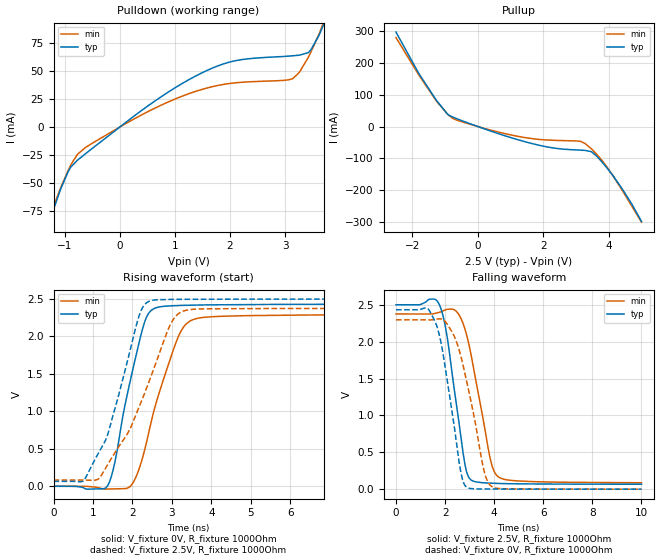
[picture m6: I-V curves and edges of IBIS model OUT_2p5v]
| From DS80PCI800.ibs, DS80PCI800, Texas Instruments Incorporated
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[Model]   OUT_2p5v
Model_type   Output
Polarity   Non-Inverting
Vmeas = 1.25
Vref = 0
Cref = 1pF
Rref = 1000000
|   typ   min   max
C_comp   1.378pF   1.280pF   1.479p
[Voltage Range]   2.5   2.375   2.625
[Temperature Range]   25   105   -40
[Pullup Reference]   2.5   2.375   2.625
[Pulldown Reference]   0   0   0
[Power Clamp Reference]   2.5   2.375   2.625
[GND Clamp Reference]   0   0   0
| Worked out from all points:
|   slope of the pulldown table from 0 to 0.375 V, typ, clamps not added: 26.8 ohm
|   slope of the pullup table from 0 to 0.375 V, typ, clamps not added: 27.5 ohm
|   falling waveform, V_fixture 2.5V, R_fixture 1000Ohm: 20-80 % time 601ps typ, 762ps min, NA max; typ from 2.5 V to 0.067 V
|   rising waveform, V_fixture 0V, R_fixture 1000Ohm: 20-80 % time 565ps typ, 749ps min, NA max; typ from 0 V to 2.43 V
|   rising waveform, V_fixture 2.5V, R_fixture 1000Ohm: 20-80 % time 777ps typ, 1.11ns min, NA max; typ from 0.065 V to 2.5 V
|   falling waveform, V_fixture 0V, R_fixture 1000Ohm: 20-80 % time 664ps typ, 842ps min, NA max; typ from 2.43 V to 0 V
[Pulldown]
|   Voltage   I(typ)   I(min)   I(max)
-2.5V     -298.7mA   -280mA     NA
-1.765V   -160.5mA   -156.1mA   NA
-1.278V   -84.06mA   -80.65mA   NA
-932.5mV  -39.33mA   -38.27mA   NA
-625mV    -23.86mA   -18.28mA   NA
1.482V    48.06mA    33.4mA     NA
2.105V    59.15mA    39.43mA    NA
3.14V     63.49mA    43.2mA     NA
3.425V    66.44mA    62.31mA    NA
3.62V     81.94mA    83.1mA     NA
3.808V    103.3mA    107mA      NA
4.992V    297.1mA    301.3mA    NA
[Pullup]
|   Voltage   I(typ)   I(min)   I(max)
-2.5V     298mA      280.7mA    NA
-1.788V   164.9mA    160.2mA    NA
-1.248V   80.21mA    78.1mA     NA
-887.5mV  36.11mA    35.28mA    NA
110mV     -4.056mA   -3.25mA    NA
1.58V     -51.78mA   -37.04mA   NA
2.353V    -68.3mA    -43.53mA   NA
3.275V    -75.25mA   -53.73mA   NA
3.47V     -79.77mA   -70.76mA   NA
3.928V    -129.1mA   -125.8mA   NA
4.468V    -206.8mA   -211.8mA   NA
4.992V    -299.3mA   -301.7mA   NA
[Ramp]
R_load = 1000
|   typ   min   max
dV/dt_r   1.4587/5.65153e-10   1.37506/7.48827e-10  NA
dV/dt_f   1.46/6.00558e-10   1.37258/7.61961e-10  NA
[Falling Waveform]
V_fixture = 2.5V
V_fixture_min = 2.375V
R_fixture = 1000Ohm
C_fixture = 0F
|   Time   V(typ)   V(min)   V(max)
0s        2.5V       2.375V     NA
1.46ns    2.577V     2.375V     NA
1.761ns   2.504V     2.397V     NA
2.071ns   2.091V     2.437V     NA
2.523ns   1.002V     2.386V     NA
2.811ns   330.9mV    2.168V     NA
3.037ns   130mV      1.856V     NA
3.826ns   82.01mV    430.7mV    NA
4.195ns   77.39mV    161mV      NA
10ns      66.51mV    87.19mV    NA
[Rising Waveform]
V_fixture = 0V
V_fixture_min = 0V
R_fixture = 1000Ohm
C_fixture = 0F
|   Time   V(typ)   V(min)   V(max)
0s        10.15uV    20.46uV    NA
1.374ns   7.664mV    -36.92mV   NA
1.555ns   319.5mV    -34.85mV   NA
1.761ns   949.3mV    -32.5mV    NA
2.027ns   1.599V     55.63mV    NA
2.322ns   2.211V     509.5mV    NA
2.574ns   2.38V      1.062V     NA
3.154ns   2.413V     1.985V     NA
3.531ns   2.418V     2.224V     NA
10ns      2.431V     2.292V     NA
[Rising Waveform]
V_fixture = 2.5V
V_fixture_min = 2.375V
R_fixture = 1000Ohm
C_fixture = 0F
|   Time   V(typ)   V(min)   V(max)
0s        65.02mV    82.67mV    NA
753.9ps   69.77mV    82.67mV    NA
1.11ns    415.7mV    89.3mV     NA
1.271ns   566.4mV    197.6mV    NA
1.946ns   1.825V     770.8mV    NA
2.175ns   2.286V     1.066V     NA
2.416ns   2.468V     1.39V      NA
2.989ns   2.495V     2.187V     NA
3.346ns   2.496V     2.348V     NA
10ns      2.5V       2.375V     NA
[Falling Waveform]
|Gnd
V_fixture = 0V
V_fixture_min = 0V
R_fixture = 1000Ohm
C_fixture = 0F
|   Time   V(typ)   V(min)   V(max)
0s        2.432V     2.295V     NA
1.271ns   2.455V     2.295V     NA
1.612ns   2.258V     2.303V     NA
1.882ns   1.901V     2.303V     NA
2.366ns   867.2mV    2.079V     NA
2.646ns   218.2mV    1.798V     NA
2.88ns    26.32mV    1.46V      NA
3.635ns   2.16mV     186.6mV    NA
3.927ns   1.896mV    30.56mV    NA
10ns      148.7uV    345.3uV    NA
